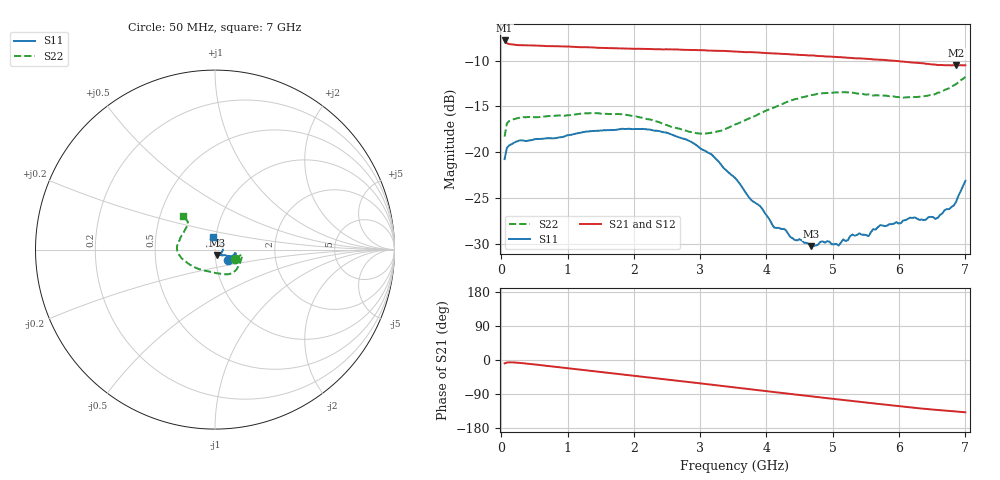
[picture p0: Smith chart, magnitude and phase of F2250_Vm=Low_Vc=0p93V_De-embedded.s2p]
! Integrated Device Technology
! Corporate Headquarters
! 6024 Silver Creek Valley Road
! San Jose, CA 95138  USA
! Phone:  1-408-284-8200
! Toll Free:  1-800-223-1366
! Webpage:  http://www.idt.com/
! Timing and RF Division
! 515 Groton Road, Suite 102
! Westford, MA 01886-6024
! Device:  F2250
! Description: Voltage Variable RF Attenuator
! Frequency:  50.0 -  6000.00 MHz
! Package:  3x3 mm Thin QFN Plastic Package: 16 pin
! Ports:  2 RF, 3 DC
!  Pin  1  = GND
!  Pin  2  = NC
!  Pin  3  = RF1  = Port 1
!  Pin  4  = NC
!  Pin  5  = GND
!  Pin  6  = GND
!  Pin  7  = GND
!  Pin  8  = GND
!  Pin  9  = NC
!  Pin 10  = RF2  = Port 2
!  Pin 11  = NC
!  Pin 12  = GND
!  Pin 13  = GND
!  Pin 14  = VCNTRL
!  Pin 15  = VDD
!  Pin 16  = VMODE
! Vcntrl:  0.930 Volts
! Vmode:  +0.000 Volts
! Vdd:  +3.30  Volts
! Current:  1.180 mA
! Data:  The device was measured on a the F2250 evaluation board which has
!  individual transmission lines to the RF pins.  Data was collected
!  using a calibrated network analyzer.  The evaluation board was
!  de-embedded using a TRL calibration technique.
!  The reference plane is the edge of the package pin.
! Misc:  SN 10
!  Action Tracker AT0258
! Date Measured:  2014-11-26
! Date:  2015-10-15  MJV
! Note:
!  Integrated Device Technology supplies this data as a sample of measured
!  data at the package pin for this product.  Your particular data for this
!  product may vary.
!  Data was taken at 25 degrees C.
!  Integrated Device Technology reserves the right to change this data at anytime.
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# GHz S dB R 50
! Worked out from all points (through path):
!   201 points, 50 MHz to 7 GHz, reference 50 ohm
!   highest |S21| = -7.82 dB at 50 MHz (marker M1); lowest = -10.5 dB at 6.861 GHz (marker M2)
!   group delay of S21, straight-line fit = 55.2 ps
!   lowest |S11| = -30.2 dB at 4.672 GHz (marker M3), VSWR 1.06, Z = 50.9 - j2.97 ohm
!   |S11| at or under -10 dB: start of sweep to end of sweep
!   |S22| runs from -18.3 to -11.8 dB; largest |S21 - S12| = 0.0012
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0.05  -20.73 -38.1  -7.82 -8.8  -7.81 -8.8  -18.28 -24.3
0.08475  -19.52 -19.3  -8.12 -6.6  -8.11 -6.6  -16.84 -13.4
0.189  -18.97 -10.9  -8.26 -6.4  -8.27 -6.4  -16.39 -10.9
1.2315  -17.80 -22.2  -8.55 -26.3  -8.54 -26.3  -15.75 -42.1
1.857  -17.46 -23.7  -8.69 -38.6  -8.69 -38.6  -15.87 -56.5
2.37825  -17.68 -22.5  -8.76 -48.9  -8.78 -48.9  -16.70 -70.1
3.0385  -19.72 -22.4  -8.88 -62.4  -8.87 -62.4  -17.98 -101.6
3.525  -22.78 -28.2  -9.02 -72.5  -9.03 -72.5  -16.98 -130.7
3.90725  -25.89 -40.1  -9.15 -80.3  -9.15 -80.3  -15.74 -149.1
4.11575  -28.20 -49.6  -9.23 -84.6  -9.22 -84.6  -15.11 -157.4
4.67175  -30.22 -71.1  -9.45 -95.9  -9.43 -95.9  -13.76 -173.1
4.7065  -30.19 -73.3  -9.45 -96.6  -9.46 -96.6  -13.74 -173.7
4.915  -29.68 -71.1  -9.57 -100.7  -9.56 -100.7  -13.53 -178.3
5.08875  -30.15 -66.8  -9.63 -104.2  -9.62 -104.2  -13.48 177.7
5.29725  -28.95 -55.3  -9.73 -108.2  -9.73 -108.2  -13.50 173.1
5.5405  -29.13 -43.7  -9.83 -113.1  -9.81 -113.1  -13.69 166.8
5.71425  -27.94 -34.2  -9.92 -116.4  -9.91 -116.4  -13.82 162.2
5.85325  -27.83 -25.6  -9.99 -119.0  -9.98 -119.1  -13.89 158.6
6.166  -27.12 -3.0  -10.19 -124.9  -10.18 -125.0  -14.00 148.5
6.54825  -27.25 39.1  -10.45 -131.4  -10.45 -131.5  -13.65 137.0
6.861  -25.37 81.5  -10.53 -135.9  -10.53 -135.9  -12.56 133.7
7  -23.11 100.8  -10.52 -138.0  -10.51 -138.1  -11.78 133.5
